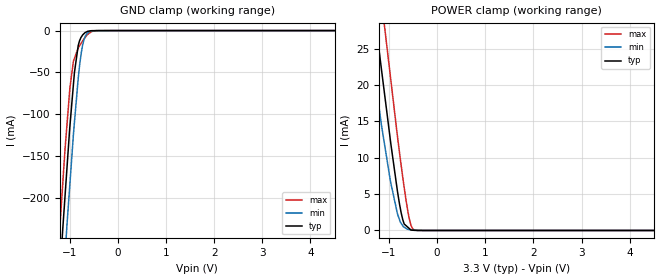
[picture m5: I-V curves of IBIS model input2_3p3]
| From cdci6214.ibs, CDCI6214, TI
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|   input2_3p3 Model
[Model]   input2_3p3
Model_type   Input
Vinl = 0.66
Vinh = 2.64
|   typ   min   max
C_comp   1.100E-12   1.095E-12   1.110E-12
|  Where Nom  PVT is Nominal Process, 3.3V,   32C
|   Fast PVT is Strong Process,  3.465V, -35C
|   Slow PVT is Weak Process,   3.135V,  110C
[Model spec]
|subparameter
Vinl   0.66   0.627   0.693
Vinh   2.64   2.508   2.772
[Voltage Range]   3.3   3.135   3.465
|Junction Temperature
[Temperature Range]   32   110   -35
[Power Clamp Reference]   3.3   3.135   3.465
[GND Clamp Reference]   0   0   0
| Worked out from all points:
|   GND clamp passes 1 mA (typ) near -0.63 V on its own axis
|   POWER clamp passes 1 mA (typ) near -0.69 V on its own axis
[GND Clamp]
|   Voltage   I(typ)   I(min)   I(max)
-3.3V     -2.319A    -2.383A    -2.269A
-1.236V   -319.7mA   -390.1mA   -261.7mA
-1.146V   -237.6mA   -310.2mA   -183mA
-1.099V   -198.9mA   -269.2mA   -142.7mA
-1.056V   -162.7mA   -230.9mA   -111.2mA
-997.7mV  -114.6mA   -183.6mA   -68.81mA
-903.5mV  -50.29mA   -110.1mA   -33.42mA
-824.3mV  -17.78mA   -56.84mA   -20.83mA
-765.4mV  -8.098mA   -28.23mA   -15.34mA
-709mV    -3.868mA   -11.71mA   -10.2mA
-626.3mV  -828uA     -2.657mA   -4.534mA
6.6V      0A         0A         0A
[POWER Clamp]
|   Voltage   I(typ)   I(min)   I(max)
-3.3V     150.6mA    135.7mA    169.2mA
-1.431V   37.45mA    28.19mA    47.96mA
-1.25V    27.33mA    19.04mA    36.99mA
-1.156V   22.16mA    14.5mA     31.69mA
-969.3mV  12.36mA    6.772mA    21.15mA
-823.8mV  5.389mA    2.287mA    12.94mA
-747.1mV  2.442mA    987.6uA    8.975mA
-683.7mV  887.5uA    450.7uA    5.899mA
-618.9mV  508uA      184.3uA    3.092mA
-538.7mV  54.68uA    58.52uA    642.1uA
-401.1mV  2.09uA     18.57uA    3.743uA
6.6V      0A         0A         0A
